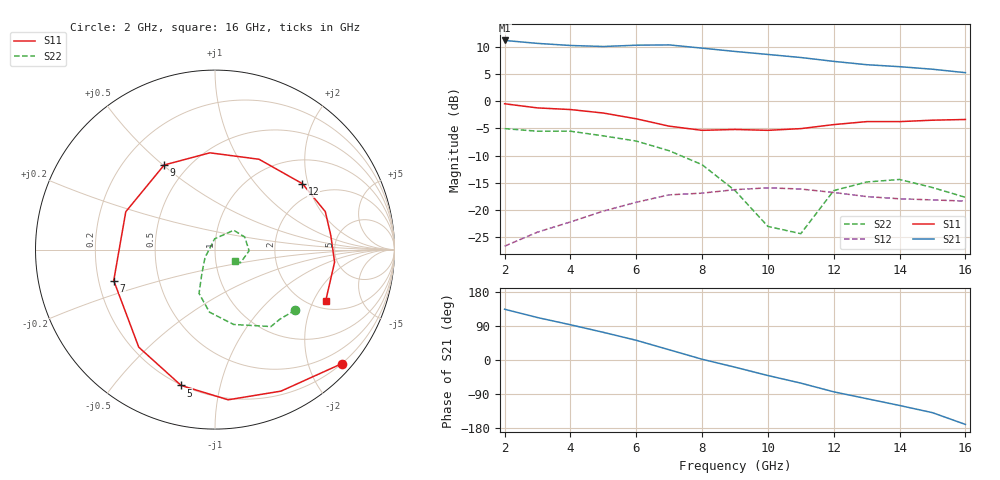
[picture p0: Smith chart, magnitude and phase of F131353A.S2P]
!ATF-13135
!S-PARAMETERS at Vds=2.5V  Id=20mA.  LAST UPDATED 07-22-92
# ghz s ma r 50
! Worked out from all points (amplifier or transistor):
!   15 points, 2 GHz to 16 GHz, reference 50 ohm
!   highest |S21| = 11.2 dB at 2 GHz (marker M1)
!   |S21| within 3 dB of that: start of sweep to 10.73 GHz
!   unconditionally stable (mu >= 1): 9.816 GHz to end of sweep
!   at 4 GHz: K = 0.60, MSG = 16.3 dB, |S12| = -22.3 dB
!   at 9 GHz: K = 0.96, MSG = 12.8 dB, |S12| = -16.3 dB
!   at 16 GHz: K = 1.34, MAG = 8.4 dB, |S12| = -18.4 dB
!   lowest NFmin = 0.40 dB at 2 GHz
!   S11 on the Smith chart (normalised r, x): 2 GHz: 0.20, -2.59; 5 GHz: 0.20, -0.76; 7 GHz: 0.26, -0.14; 9 GHz: 0.37, +0.50; 12 GHz: 1.58, +1.85; 16 GHz: 2.34, -2.50
2  0.95 -42.0  3.65 134.0  0.046 62.0  0.56 -37.0
3  0.87 -65.0  3.43 112.0  0.062 40.0  0.53 -47.0
4  0.84 -85.0  3.28 93.0  0.077 31.0  0.53 -54.0
5  0.78 -104.0  3.21 73.0  0.097 18.0  0.48 -62.0
6  0.69 -128.0  3.3 52.0  0.117 7.0  0.43 -76.0
7  0.59 -163.0  3.32 27.0  0.137 -12.0  0.35 -95.0
8  0.54 157.0  3.1 2.0  0.142 -27.0  0.26 -110.0
9  0.55 121.0  2.89 -19.0  0.153 -43.0  0.15 -119.0
10  0.54 93.0  2.71 -41.0  0.159 -58.0  0.07 -142.0
11  0.56 64.0  2.54 -61.0  0.155 -73.0  0.06 92.0
12  0.61 37.0  2.34 -84.0  0.144 -89.0  0.15 46.0
13  0.65 19.0  2.18 -102.0  0.132 -100.0  0.18 23.0
14  0.65 7.0  2.09 -120.0  0.126 -114.0  0.19 -2.0
15  0.67 -6.0  1.98 -139.0  0.123 -119.0  0.16 -27.0
16  0.68 -25.0  1.84 -170.0  0.12 -134.0  0.13 -30.0
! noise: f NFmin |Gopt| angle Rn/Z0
2  0.4  0.75  34  0.26
4  0.5  0.58  87  0.22
6  0.8  0.47  130  0.18
8  1  0.37  -163  0.17
10  1.1  0.42  -114  0.41
12  1.2  0.47  -65  0.8
14  1.4  0.52  -15  1.2
